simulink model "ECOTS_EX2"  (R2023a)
settings: Solver=ode23tb  StartTime=0.0  StopTime=meas.Time(end)  RelTol=1e-3
libraries: component_lib x8

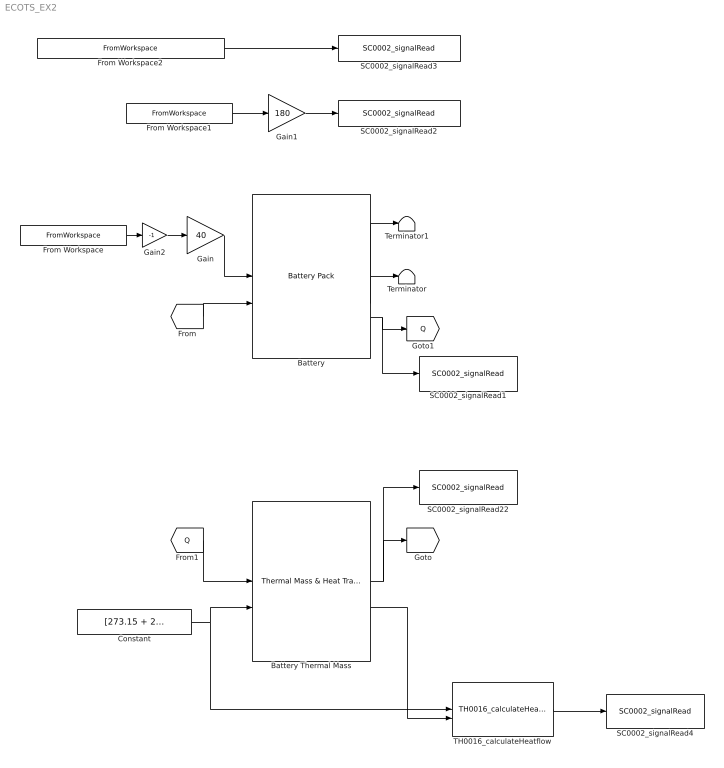
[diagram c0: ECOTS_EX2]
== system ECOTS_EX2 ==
  Battery : component_lib/Battery Pack  SOC_0=1  Nx=40  Ny=180
  Battery Thermal Mass : component_lib/Thermal Mass & Heat Transfer  n=100  d=10e-3  L=4  m=40 * 180 * 0.048  cp=1040  T_0=273 + 25
  Constant : Constant  Value=[273.15 + 20; 1e5; 0.05]
  From Workspace : FromWorkspace  VariableName=[meas.Time, meas.Current]
  From Workspace1 : FromWorkspace  VariableName=[meas.Time, meas.Voltage]
  From Workspace2 : FromWorkspace  VariableName=[meas.Time, meas.Battery_Temp_degC + 273.15]
  Gain : Gain  Gain=40
  Gain1 : Gain  Gain=180
  Gain2 : Gain  Gain=-1
  SC0002_signalRead1 : component_lib/Data & Control/SC0002_signalRead  SigName=generatedHeat
  SC0002_signalRead2 : component_lib/Data & Control/SC0002_signalRead  SigName=measuredBatteryVoltage
  SC0002_signalRead22 : component_lib/Data & Control/SC0002_signalRead  SigName=batteryTemperature
  SC0002_signalRead3 : component_lib/Data & Control/SC0002_signalRead  SigName=measuredBatteryTemperature
  SC0002_signalRead4 : component_lib/Data & Control/SC0002_signalRead  SigName=batteryCooling
  TH0016_calculateHeatflow : component_lib/Thermal Systems/TH0016_calculateHeatflow
  Terminator : Terminator
  Terminator1 : Terminator
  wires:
  Battery/2 -> Terminator/1
  Battery/1 -> Terminator1/1
  Constant/1 -> TH0016_calculateHeatflow/1, Battery Thermal Mass/2
  Battery Thermal Mass/1 -> SC0002_signalRead22/1, [T]
  [T] -> Battery/2
  Battery/3 -> SC0002_signalRead1/1, [Q]
  [Q] -> Battery Thermal Mass/1
  Gain1/1 -> SC0002_signalRead2/1
  From Workspace1/1 -> Gain1/1
  Gain/1 -> Battery/1
  Gain2/1 -> Gain/1
  From Workspace/1 -> Gain2/1
  From Workspace2/1 -> SC0002_signalRead3/1
  TH0016_calculateHeatflow/1 -> SC0002_signalRead4/1
  Battery Thermal Mass/2 -> TH0016_calculateHeatflow/2
